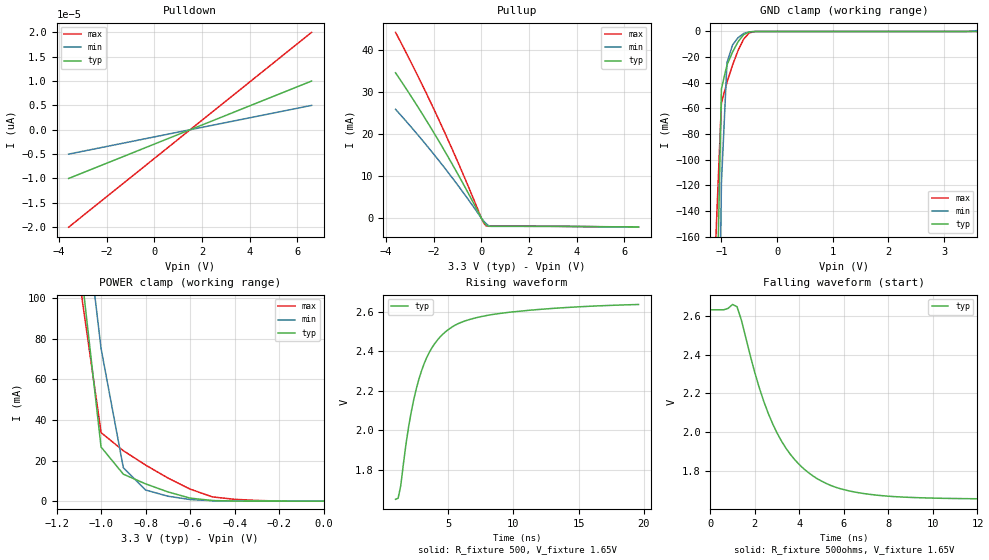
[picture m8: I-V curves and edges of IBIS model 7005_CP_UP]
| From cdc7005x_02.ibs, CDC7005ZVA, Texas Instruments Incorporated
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| CHARGE PUMP OUT FOR PULL-UP PULSE
[Model]   7005_CP_UP
Model_type   3-state
Polarity   Non-Inverting
Enable   Active-High
Vmeas = 2.475V   |Vref for timing measurements.
Cref = 0pF   |load capacitance for timing spec.
Rref = 500ohms   |500 Ohm to VCC/2
Vref = 1.65V   |Timing specification test load voltage; GND
|   typ   min   max
C_comp   2.86pF   2.8pF   2.91pF
[Temperature range]   27   125   -20
[Voltage range]   3.3   3.0   3.6
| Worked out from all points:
|   slope of the pullup table from 0 to 0.495 V, typ, clamps not added: 250 ohm
|   GND clamp passes 1 mA (typ) near -0.53 V on its own axis
|   POWER clamp passes 1 mA (typ) near -0.56 V on its own axis
|   rising waveform, R_fixture 500, V_fixture 1.65V: 20-80 % time 2.38ns typ, NA min, NA max; typ from 1.65 V to 2.64 V
|   falling waveform, R_fixture 500ohms, V_fixture 1.65V: 20-80 % time 2.16ns typ, NA min, NA max; typ from 2.63 V to 1.66 V
| Notes: (1) Vtable = Vcc - Voutput
|   (2) Pullup data includes the effects of the ESD
|   clamping circuitry
[Pullup]
|   27C:3.3V:nominal   125C:3.0V:weak   -20C:3.6V:strong
|  Voltage   I(typ)   I(min)   I(max)
-3.6V     34.63mA    25.92mA    44.28mA
-2.7V     26.83mA    20.07mA    34.29mA
-1.9V     19.46mA    14.55mA    24.86mA
-900mV    9.598mA    7.165mA    12.25mA
0V        245.2pA    1.646nA    229.1pA
100mV     -951.4uA   -726.9uA   -1.175mA
200mV     -1.669mA   -1.335mA   -1.867mA
300mV     -1.975mA   -1.784mA   -1.871mA
400mV     -1.976mA   -1.98mA    -1.875mA
6.6V      -2.136mA   -2.181mA   -2.177mA
[Pulldown]  | Is off for PULL-UP PULSE
|   27C:3.3V:nominal   125C:3.0V:weak   -20C:3.6V:strong
|  Voltage   I(typ)   I(min)   I(max)
-3.6V     -10pA      -5pA       -20pA
6.6V      10pA       5pA        20pA
[POWER Clamp]
|   27C:3.3V:nominal   125C:3.0V:weak   -20C:3.6V:strong
|  Voltage   I(typ)   I(min)   I(max)
-3.6V     3.248A     2.572A     4.171A
-1.1V     124.2mA    167.9mA    110.9mA
-1V       26.63mA    75.14mA    33.74mA
-900mV    13.27mA    16.44mA    24.83mA
-800mV    8.502mA    5.477mA    17.76mA
-700mV    4.551mA    2.43mA     11.4mA
-600mV    1.477mA    777.7uA    5.912mA
-500mV    299.3uA    201uA      2.081mA
-400mV    26.9uA     28.19uA    894.9uA
-300mV    1.191uA    2.625uA    331.3uA
0V        245.2pA    1.646nA    229.2pA
[GND Clamp]
|   27C:3.3V:nominal   125C:3.0V:weak   -20C:3.6V:strong
|  Voltage   I(typ)   I(min)   I(max)
-3.6V     -12.74A    -10.05A    -16.37A
-1.1V     -253.9mA   -443mA     -161.5mA
-1V       -44.77mA   -118.5mA   -55.73mA
-900mV    -26.11mA   -24.29mA   -39.68mA
-800mV    -16.07mA   -10.54mA   -26.23mA
-700mV    -7.95mA    -4.789mA   -14.73mA
-600mV    -2.456mA   -1.484mA   -5.897mA
-500mV    -327.7uA   -267.2uA   -1.086mA
-400mV    -21.87uA   -33.38uA   -64.02uA
3.3V      245.2pA    2.625uA    -48.88nA
3.6V      1.191uA    777.7uA    229.2pA
[ramp]
| variable   typ   min   max
dV/dt_r   0.5931/2.3962E-09   NA   NA
dV/dt_f   0.5931/2.1882E-09   NA   NA
[Rising Waveform]
R_fixture = 500
V_fixture =  1.65V
|   27C:3.3V:nominal   125C:3.0V:weak  -20C:3.6V:strong
|   Time   V(typ)   V(min)   V(max)
952ps     1.65V      NA         NA
1.15ns    1.656V     NA         NA
1.35ns    1.718V     NA         NA
1.95ns    2.015V     NA         NA
2.75ns    2.26V      NA         NA
3.75ns    2.418V     NA         NA
4.95ns    2.507V     NA         NA
6.35ns    2.554V     NA         NA
8.95ns    2.591V     NA         NA
19.6ns    2.636V     NA         NA
[Falling Waveform]
R_fixture = 500ohms
V_fixture =  1.65V
V_fixture_min = 1.5V
V_fixture_max = 1.8V   | 1.8V will remove the warning. Plot was truncated to
|   allow faster simulation periodes.
|   27C:3.3V:nominal   125C:3.0V:weak -20C:3.6V:strong
|   Time   V(typ)   V(min)   V(max)
0s        2.631V     NA         NA
1.2ns     2.647V     NA         NA
2.2ns     2.23V      NA         NA
2.6ns     2.099V     NA         NA
3ns       1.996V     NA         NA
4ns       1.834V     NA         NA
5.4ns     1.727V     NA         NA
6.8ns     1.686V     NA         NA
8.8ns     1.666V     NA         NA
19.6ns    1.655V     NA         NA
